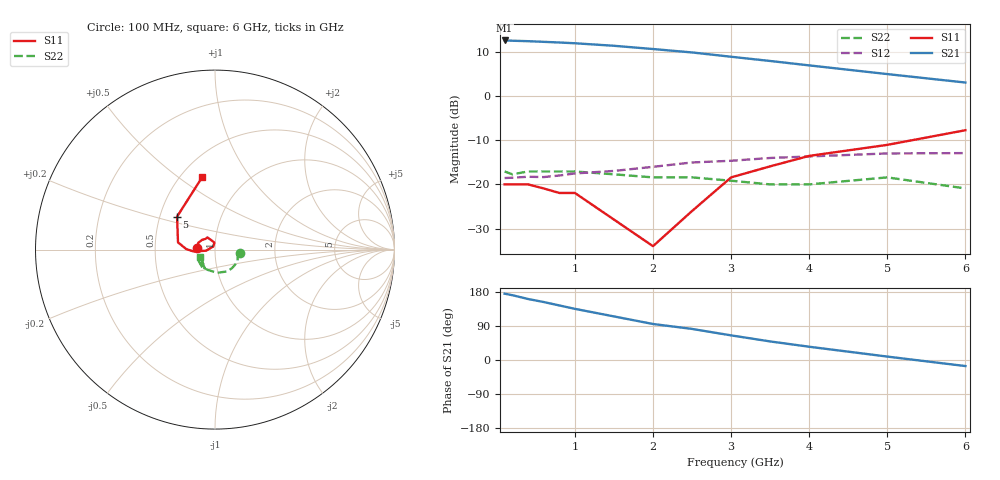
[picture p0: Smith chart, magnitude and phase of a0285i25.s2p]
!  MSA-0285 S AND NOISE PARAMETERS
!  Id=25mA  LAST UPDATED 07-22-92
# ghz s ma r 50
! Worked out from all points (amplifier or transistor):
!   14 points, 100 MHz to 6 GHz, reference 50 ohm
!   highest |S21| = 12.6 dB at 100 MHz (marker M1)
!   |S21| within 3 dB of that: start of sweep to 2.648 GHz
!   unconditionally stable (mu >= 1): start of sweep to end of sweep
!   at 400 MHz: K = 1.20, MAG = 12.7 dB, |S12| = -18.3 dB
!   at 2 GHz: K = 1.19, MAG = 10.7 dB, |S12| = -16.0 dB
!   at 6 GHz: K = 1.42, MAG = 4.2 dB, |S12| = -12.9 dB
!   lowest NFmin = 6.00 dB at 100 MHz
!   S11 on the Smith chart (normalised r, x): 100 MHz: 0.82, +0.02; 5 GHz: 0.61, +0.24; 6 GHz: 0.63, +0.62
0.1  0.1 174.0  4.25 175.0  0.118 2.0  0.14 -7.0
0.2  0.1 168.0  4.22 171.0  0.119 3.0  0.13 -12.0
0.4  0.1 157.0  4.17 161.0  0.122 6.0  0.14 -26.0
0.6  0.09 143.0  4.1 153.0  0.121 7.0  0.14 -38.0
0.8  0.08 132.0  4.03 144.0  0.126 11.0  0.14 -48.0
1  0.08 122.0  3.95 135.0  0.133 12.0  0.14 -60.0
1.5  0.04 95.0  3.7 115.0  0.142 16.0  0.13 -85.0
2  0.02 117.0  3.4 95.0  0.158 17.0  0.12 -110.0
2.5  0.05 -173.0  3.11 82.0  0.177 20.0  0.12 -128.0
3  0.12 -175.0  2.78 65.0  0.185 19.0  0.11 -148.0
3.5  0.16 179.0  2.49 49.0  0.199 14.0  0.1 -145.0
4  0.21 169.0  2.22 35.0  0.207 11.0  0.1 -134.0
5  0.28 139.0  1.77 9.0  0.224 4.0  0.12 -118.0
6  0.41 100.0  1.42 -16.0  0.226 -5.0  0.09 -154.0
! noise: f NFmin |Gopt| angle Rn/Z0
0.1  6  0.09  0  1.15
0.5  6.3  0.08  3  1.15
1  6.5  0.07  3  1.14
2  6.9  0.05  -2  1.1
